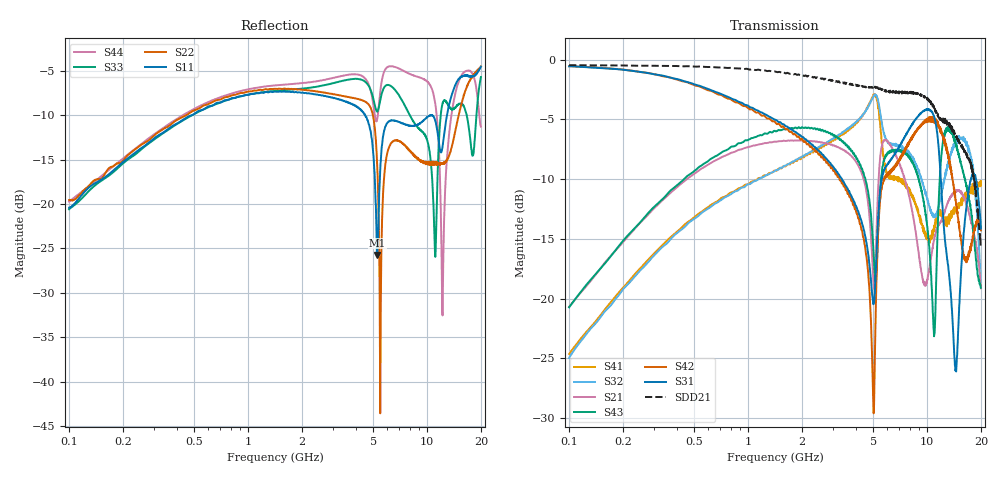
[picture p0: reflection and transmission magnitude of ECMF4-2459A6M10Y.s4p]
!ECMF4-2459A6M10Y
!P1 -@@@@@@@- P3
!P2 -@@@@@@@- P4
!Typical device
!21/10/2019 12:08:55
!Probes on PCB
!P1 Probe Type : T26D-GSGSG200 ; Probe S/N : 18A240
!P2 Probe Type : T26D-GSGSG200 ; Probe S/N : 18A240
!P3 Probe Type : T26D-GSGSG200 ; Probe S/N : 18A241
!P4 Probe Type : T26D-GSGSG200 ; Probe S/N : 18A241
!Instrument Manufacturer :Agilent Technologies
!Instrument Model : E8362B
!Instrument Serial Number : MY43020422
!Instrument Firmware Rev : A.06.04.32
!Start Freq : 1,00e+08 ; Stop Freq : 2,00e+10
!Ports power : -12 dBm ; IFBW : 1,00e+02 Hz
!Calibration kit : 129-240 (257440)
!Prober : PM8
!Darkness measurement : False
!Voltage measurement : False
!Temperature measurement : Tamb=26°C
!Lane#1 or #2
# Hz S  RI  R 50
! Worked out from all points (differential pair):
!   1601 points, 100 MHz to 20 GHz, reference 50 ohm
!   strongest paths, dB at 100 MHz, 376.1 MHz, 1.414 GHz, 5.318 GHz, 20 GHz:
!     S31: -0.6, -1.5, -5.0, -13.6, -14.1
!     S42: -0.6, -1.6, -5.2, -14.9, -14.3
!     S43: -20.7, -10.8, -6.0, -14.7, -19.1
!     S21: -20.7, -11.0, -6.9, -11.1, -19.1
!     S32: -25.0, -14.9, -9.3, -3.3, -18.6
!     S41: -24.6, -14.7, -9.3, -3.9, -10.2
!   taken as a pair (ports 1,2 in; 3,4 out), SDD21 dB: -0.5, -0.5, -1.0, -2.4, -15.7
!   lowest |S11| = -25.7 dB at 5.266 GHz (marker M1), VSWR 1.11, Z = 49.2 + j5.07 ohm
!   |S11| at or under -10 dB: start of sweep to 484.9 MHz; 4.515 GHz to 10.44 GHz (5.926 GHz wide, 79.2 % of centre); 10.71 GHz to 12.93 GHz (2.221 GHz wide, 18.8 % of centre)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
1e8  0.0648 0.0698  0.0222 0.089  0.929 -0.1281  -0.0166 -0.0563
     0.023 0.0894  0.0765 0.0722  -0.0172 -0.0552  0.9277 -0.1324
     0.922 -0.1655  -0.0169 -0.0538  0.0635 0.0684  0.0224 0.0892
     -0.0163 -0.0564  0.9292 -0.1323  0.0205 0.0897  0.0645 0.0804
2.661953e9  0.248 -0.3205  0.4124 -0.1728  -0.1121 -0.3789  0.1458 0.4153
            0.4142 -0.1717  0.2436 -0.3463  0.1607 0.4166  -0.1174 -0.3665
            -0.1086 -0.3774  0.1583 0.4136  0.4522 -0.1172  0.4644 -0.1886
            0.1395 0.4128  -0.1128 -0.3632  0.4646 -0.1872  0.484 -0.1246
5.265724e9  -0.0058 0.0514  0.2294 0.0227  -0.1701 -0.0337  0.4883 -0.4549
            0.229 0.021  -0.165 0.0179  0.5705 -0.3775  -0.1076 -0.1021
            -0.1722 -0.0363  0.5869 -0.3719  0.2003 -0.2642  0.1521 -0.00556
            0.5064 -0.4498  -0.1061 -0.1072  0.152 -0.00436  0.2414 -0.1776
1.109278e10  0.1201 0.271  0.1285 0.1259  -0.00835 -0.5314  -0.1569 -0.1183
             0.1355 0.1234  -0.1412 0.0888  -0.1265 0.1757  0.1466 -0.5225
             -0.0159 -0.5563  -0.1341 0.1772  0.00276 -0.0511  0.0642 -0.0472
             -0.1734 -0.1127  0.1334 -0.5445  0.0621 -0.0506  -0.3607 -0.1013
1.225137e10  0.0988 0.1904  0.2165 0.0422  -0.1633 -0.1427  -0.095 0.1881
             0.2164 0.0368  -0.0889 0.1453  0.1747 0.2154  -0.2044 -0.4207
             -0.1725 -0.1516  0.179 0.2345  0.1303 -0.3462  0.2526 -0.3916
             -0.0981 0.189  -0.1921 -0.4338  0.2411 -0.3743  0.0305 0.00436
1.440966e10  0.4576 0.1048  0.2531 -0.1329  -0.0327 0.0339  0.2187 -0.0518
             0.2388 -0.1426  0.0583 0.2524  0.3005 -0.2885  -0.2315 0.053
             -0.0318 0.0386  0.319 -0.322  -0.1561 -0.3141  -0.3976 -0.1968
             0.2288 -0.0658  -0.2527 0.0563  -0.3939 -0.209  -0.0198 -0.4212
2e10  0.051 -0.59  -0.0885 -0.0643  -0.1057 -0.1826  -0.2873 -0.2276
      -0.0858 -0.0697  0.197 -0.5623  -0.0969 0.0825  -0.0135 -0.2297
      -0.0921 -0.1737  -0.088 0.0774  0.1304 -0.502  0.0989 0.0738
      -0.2389 -0.1985  -0.0174 -0.1923  0.0901 0.0649  0.237 0.1351
